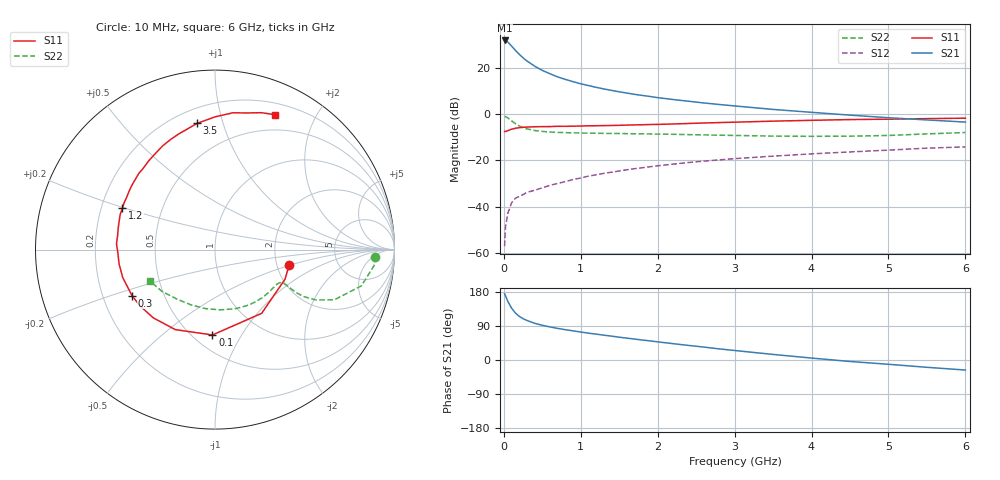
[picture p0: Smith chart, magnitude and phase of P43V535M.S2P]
! SIEMENS Small Signal Semiconductors
! BFP182
! Si NPN RF Bipolar Junction Transistor in SOT143
! VCE = 3.5 V  IC = 35 mA
! Common Emitter S-Parameters:  March  1996
# GHz  S  MA  R  50
!  f  S11  S21  S12  S22
! GHz  MAG  ANG  MAG  ANG  MAG  ANG  MAG  ANG
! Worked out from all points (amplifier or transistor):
!   36 points, 10 MHz to 6 GHz, reference 50 ohm
!   highest |S21| = 31.9 dB at 10 MHz (marker M1)
!   |S21| within 3 dB of that: start of sweep to 116 MHz
!   unconditionally stable (mu >= 1): start of sweep to 14.26 MHz; 376.9 MHz to end of sweep
!   at 250 MHz: K = 0.80, MSG = 29.6 dB, |S12| = -34.8 dB
!   at 1.4 GHz: K = 1.44, MAG = 13.8 dB, |S12| = -25.1 dB
!   at 6 GHz: K = 1.03, MAG = 4.3 dB, |S12| = -14.1 dB
!   S11 on the Smith chart (normalised r, x): 10 MHz: 2.34, -0.48; 100 MHz: 0.62, -0.76; 300 MHz: 0.33, -0.23; 1.2 GHz: 0.29, +0.20; 3.5 GHz: 0.29, +0.83; 6 GHz: 0.32, +1.49
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0.01  0.4222 -11.6  39.56 174.7  0.0014 76.0  0.8936 -2.5
0.02  0.4236 -22.9  39.47 170.0  0.0035 70.8  0.8909 -5.7
0.05  0.4401 -53.8  36.81 155.4  0.007 74.2  0.8405 -13.9
0.1  0.4758 -91.7  29.99 137.0  0.0121 59.0  0.7215 -22.8
0.15  0.4977 -116.4  24.21 124.1  0.0152 52.8  0.6265 -26.6
0.2  0.5126 -132.1  19.87 115.3  0.0167 50.7  0.5591 -27.9
0.25  0.5226 -143.1  16.63 109.0  0.0183 50.6  0.5145 -27.9
0.3  0.5286 -151.0  14.23 104.4  0.0204 51.8  0.4835 -27.4
0.4  0.5371 -163.1  11 96.9  0.0227 53.1  0.4459 -26.5
0.5  0.5403 -171.3  8.899 91.6  0.0256 53.9  0.4257 -26.2
0.6  0.5415 -178.0  7.525 87.2  0.0291 55.5  0.414 -26.4
0.7  0.5499 176.6  6.43 83.4  0.0318 57.8  0.4055 -27.0
0.8  0.5481 171.8  5.684 79.9  0.035 58.1  0.4011 -27.9
1.1  0.5634 159.7  4.181 70.8  0.046 59.1  0.3908 -31.7
1.2  0.5649 155.9  3.826 68.3  0.049 58.8  0.3881 -33.2
1.7  0.5889 140.3  2.699 55.2  0.0665 57.1  0.3784 -41.9
2.2  0.6173 126.7  2.086 43.1  0.0834 53.7  0.3686 -52.1
2.8  0.6614 112.0  1.629 29.3  0.1031 48.5  0.352 -65.9
3.5  0.7103 98.1  1.274 14.7  0.1242 42.1  0.3371 -84.6
4.5  0.7685 82.6  0.958 -3.9  0.1532 33.2  0.3359 -113.8
5.5  0.8053 71.3  0.754 -19.3  0.185 24.2  0.3762 -141.7
6  0.822 66.2  0.678 -26.5  0.197 18.9  0.403 -154.4
